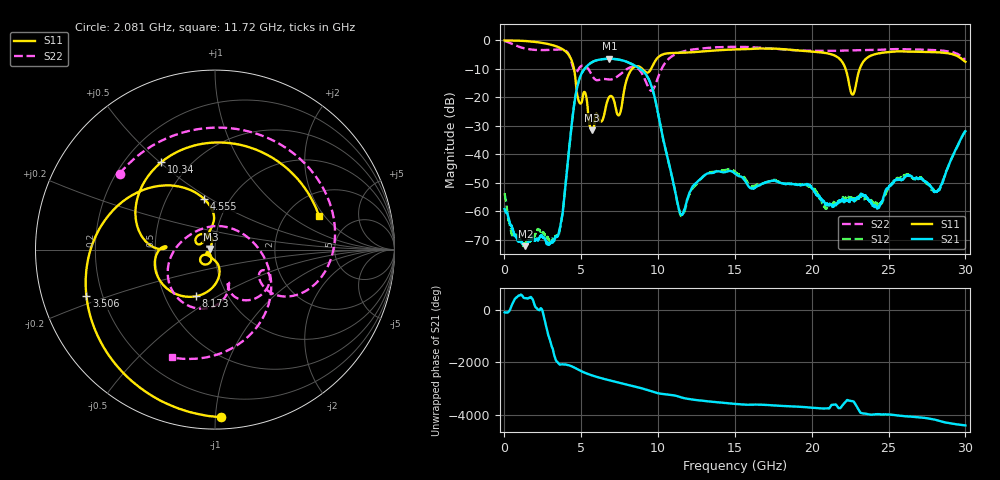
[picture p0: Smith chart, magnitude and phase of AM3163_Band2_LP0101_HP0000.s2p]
!Agilent Technologies,E8364B,MY43040894,A.07.50.67
!Agilent E8364B: A.07.50.67
!Date: Thursday, August 20, 2020 12:05:43
!Correction: S11(Full 2 Port(1,2))
!S21(Full 2 Port(1,2))
!S12(Full 2 Port(1,2))
!S22(Full 2 Port(1,2))
!S2P File: Measurements: S11, S21, S12, S22:
# Hz S  dB  R 50
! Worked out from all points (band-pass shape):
!   3201 points, 10 MHz to 30 GHz, reference 50 ohm
!   highest |S21| = -6.44 dB at 6.833 GHz (marker M1); lowest = -72.3 dB at 1.36 GHz (marker M2)
!   |S21| within 3 dB of the highest: 5.297 GHz to 8.683 GHz (3.386 GHz wide, 48.4 % of centre)
!   lowest |S11| = -31.6 dB at 5.708 GHz (marker M3), VSWR 1.05, Z = 47.5 + j0.277 ohm
!   |S11| at or under -10 dB: 4.526 GHz to 8.305 GHz (3.779 GHz wide, 58.9 % of centre); 8.97 GHz to 9.539 GHz (569.1 MHz wide, 6.15 % of centre); 22.2 GHz to 23.12 GHz (919.4 MHz wide, 4.06 % of centre)
!   |S22| runs from -17.7 to -0.3 dB; largest |S21 - S12| = 0.0036
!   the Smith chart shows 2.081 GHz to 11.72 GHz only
!   S11 on the Smith chart (normalised r, x): 2.081 GHz: 0.07, -1.03; 3.506 GHz: 0.14, -0.17; 4.555 GHz: 0.76, +0.47; 8.173 GHz: 0.71, -0.40; 10.34 GHz: 0.35, +0.51; 11.72 GHz: 2.95, +1.78
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1e7  -0.02 -3.0  -59.22 -96.1  -53.61 49.8  -0.25 -10.4
6.004281e8  -0.06 -24.7  -67.29 -29.4  -68.54 174.5  -1.51 -83.8
1.35955e9  -0.22 -56.6  -72.25 85.8  -71.32 124.1  -2.86 -161.6
2.081184e9  -0.59 -87.9  -69.68 76.4  -66.84 105.6  -3.36 141.5
3.505709e9  -2.36 -160.0  -68.22 133.1  -68.58 -8.4  -3.17 40.6
4.555359e9  -10.85 101.9  -21.85 -37.4  -21.86 -37.7  -10.63 -33.0
5.014581e9  -21.82 153.7  -11.68 -177.4  -11.69 -177.7  -8.95 -32.4
5.7081e9  -31.61 173.6  -7.62 26.2  -7.63 26.1  -12.34 -70.5
6.832725e9  -19.78 -126.6  -6.44 -159.3  -6.45 -159.4  -13.76 -70.4
7.470012e9  -26.18 -114.0  -6.76 108.9  -6.79 108.8  -12.19 -73.5
8.172903e9  -11.01 -112.4  -8.00 9.7  -8.01 9.8  -9.48 -101.2
1.000979e10  -5.90 150.1  -26.00 67.4  -25.89 66.4  -12.81 6.2
1.033781e10  -4.86 121.6  -34.88 38.7  -34.82 37.2  -8.89 -29.6
1.171547e10  -4.31 18.1  -59.29 -121.0  -60.08 -123.9  -3.77 -111.9
1.335555e10  -3.69 -73.3  -46.55 114.0  -46.36 117.9  -2.57 -171.4
1.5005e10  -3.14 -143.2  -46.82 22.9  -46.08 23.0  -2.25 132.3
1.77041e10  -2.92 94.2  -49.55 -42.5  -49.34 -45.7  -3.01 30.6
2.000958e10  -3.94 -28.2  -51.94 -121.2  -51.56 -126.7  -3.64 -50.9
2.266182e10  -19.02 -107.7  -55.89 125.3  -55.58 -89.2  -3.51 -125.8
2.500479e10  -4.13 -151.5  -51.44 -16.1  -51.50 -19.1  -3.21 176.6
2.818186e10  -4.18 107.8  -52.87 118.9  -52.78 114.4  -3.45 91.5
3e10  -7.51 38.3  -31.90 -76.7  -31.83 -77.4  -6.81 35.5
